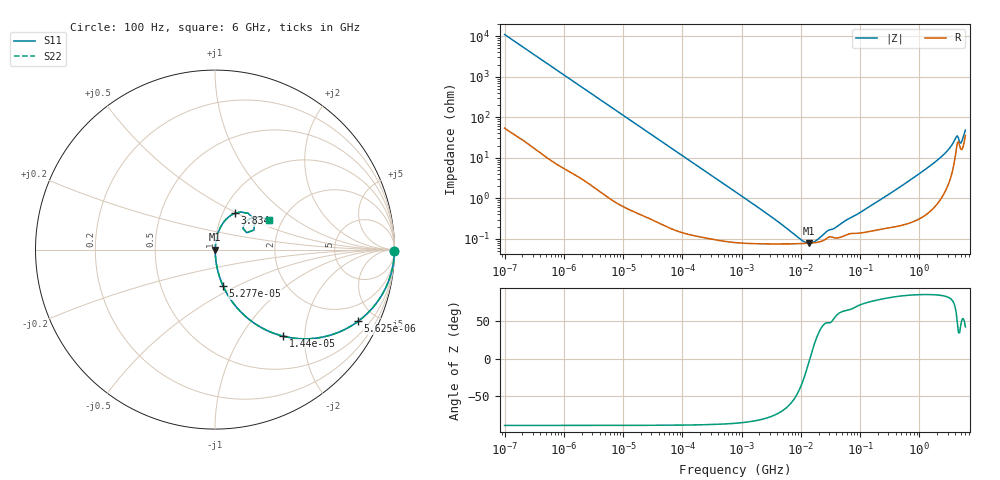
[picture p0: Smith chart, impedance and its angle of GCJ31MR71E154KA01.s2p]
!Murata Part Number: GCJ31MR71E154KA01
!These Parameters are Measured in Series Mode Connection
!Data Generated on Mar 13, 2026
!  o--ll--o
!Port1  Port2
!  o------o
!Operation Temp=25[degC], DC Bias Voltage=0[V]
!Freq. Start=100[Hz] Stop=6[GHz] 401[Steps]
# Hz S RI R 50
!Freq.(Hz) S11(Real) S11(Imag) S21(Real) S21(Imag) S12(Real) S12(Imag) S22(Real) S22(Imag)
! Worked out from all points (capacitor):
!   401 points, 100 Hz to 6 GHz, reference 50 ohm
!   read as one part in series: C = 144 nF near 109 Hz
!   lowest |Z| = 78.2 mohm at 13.6 MHz (marker M1)
!   series resonance near 14.24 MHz, so ESL is about 870 pH
!   S11 on the Smith chart (normalised r, x): 100 Hz: open; 5.625 kHz: 1.02, -3.99; 14.4 kHz: 1.01, -1.56; 52.77 kHz: 1.00, -0.43; 3.834 GHz: 1.14, +0.48; 6 GHz: 1.71, +0.65
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100  0.9999 -0.00903  0.000126 0.00903  0.000126 0.00903  0.9999 -0.00903
600  0.9969 -0.0537  0.00314 0.0537  0.00314 0.0537  0.9969 -0.0537
2008  0.9678 -0.1738  0.0322 0.1738  0.0322 0.1738  0.9678 -0.1738
5625  0.7976 -0.3992  0.2024 0.3992  0.2024 0.3992  0.7976 -0.3992
9204  0.5974 -0.4877  0.4026 0.4877  0.4026 0.4877  0.5974 -0.4877
14402  0.3791 -0.4821  0.6209 0.4821  0.6209 0.4821  0.3791 -0.4821
23569  0.1875 -0.3867  0.8125 0.3867  0.8125 0.3867  0.1875 -0.3867
40335  0.0745 -0.2583  0.9255 0.2583  0.9255 0.2583  0.0745 -0.2583
52766  0.0456 -0.2039  0.9544 0.2039  0.9544 0.2039  0.0456 -0.2039
154540  0.00654 -0.0728  0.9935 0.0728  0.9935 0.0728  0.00654 -0.0728
774597  0.00102 -0.0147  0.999 0.0147  0.999 0.0147  0.00102 -0.0147
9941735  0.000761 -0.000592  0.9992 0.000592  0.9992 0.000592  0.000761 -0.000592
1.360128e7  0.000778 -7.4e-05  0.9992 7.4e-05  0.9992 7.4e-05  0.000778 -7.4e-05
1.555665e7  0.00079 0.000145  0.9992 -0.000145  0.9992 -0.000145  0.00079 0.000145
2.784235e7  0.00104 0.00115  0.999 -0.00115  0.999 -0.00115  0.00104 0.00115
3.124326e8  0.00203 0.0126  0.998 -0.0126  0.998 -0.0126  0.00203 0.0126
1.873145e9  0.0126 0.0783  0.9874 -0.0783  0.9874 -0.0783  0.0126 0.0783
3.065283e9  0.043 0.1454  0.957 -0.1454  0.957 -0.1454  0.043 0.1454
3.8344e9  0.1097 0.202  0.8903 -0.202  0.8903 -0.202  0.1097 0.202
4.193612e9  0.1845 0.2024  0.8155 -0.2024  0.8155 -0.2024  0.1845 0.2024
5.016141e9  0.156 0.1178  0.844 -0.1178  0.844 -0.1178  0.156 0.1178
6e9  0.3029 0.1673  0.6971 -0.1673  0.6971 -0.1673  0.3029 0.1673
